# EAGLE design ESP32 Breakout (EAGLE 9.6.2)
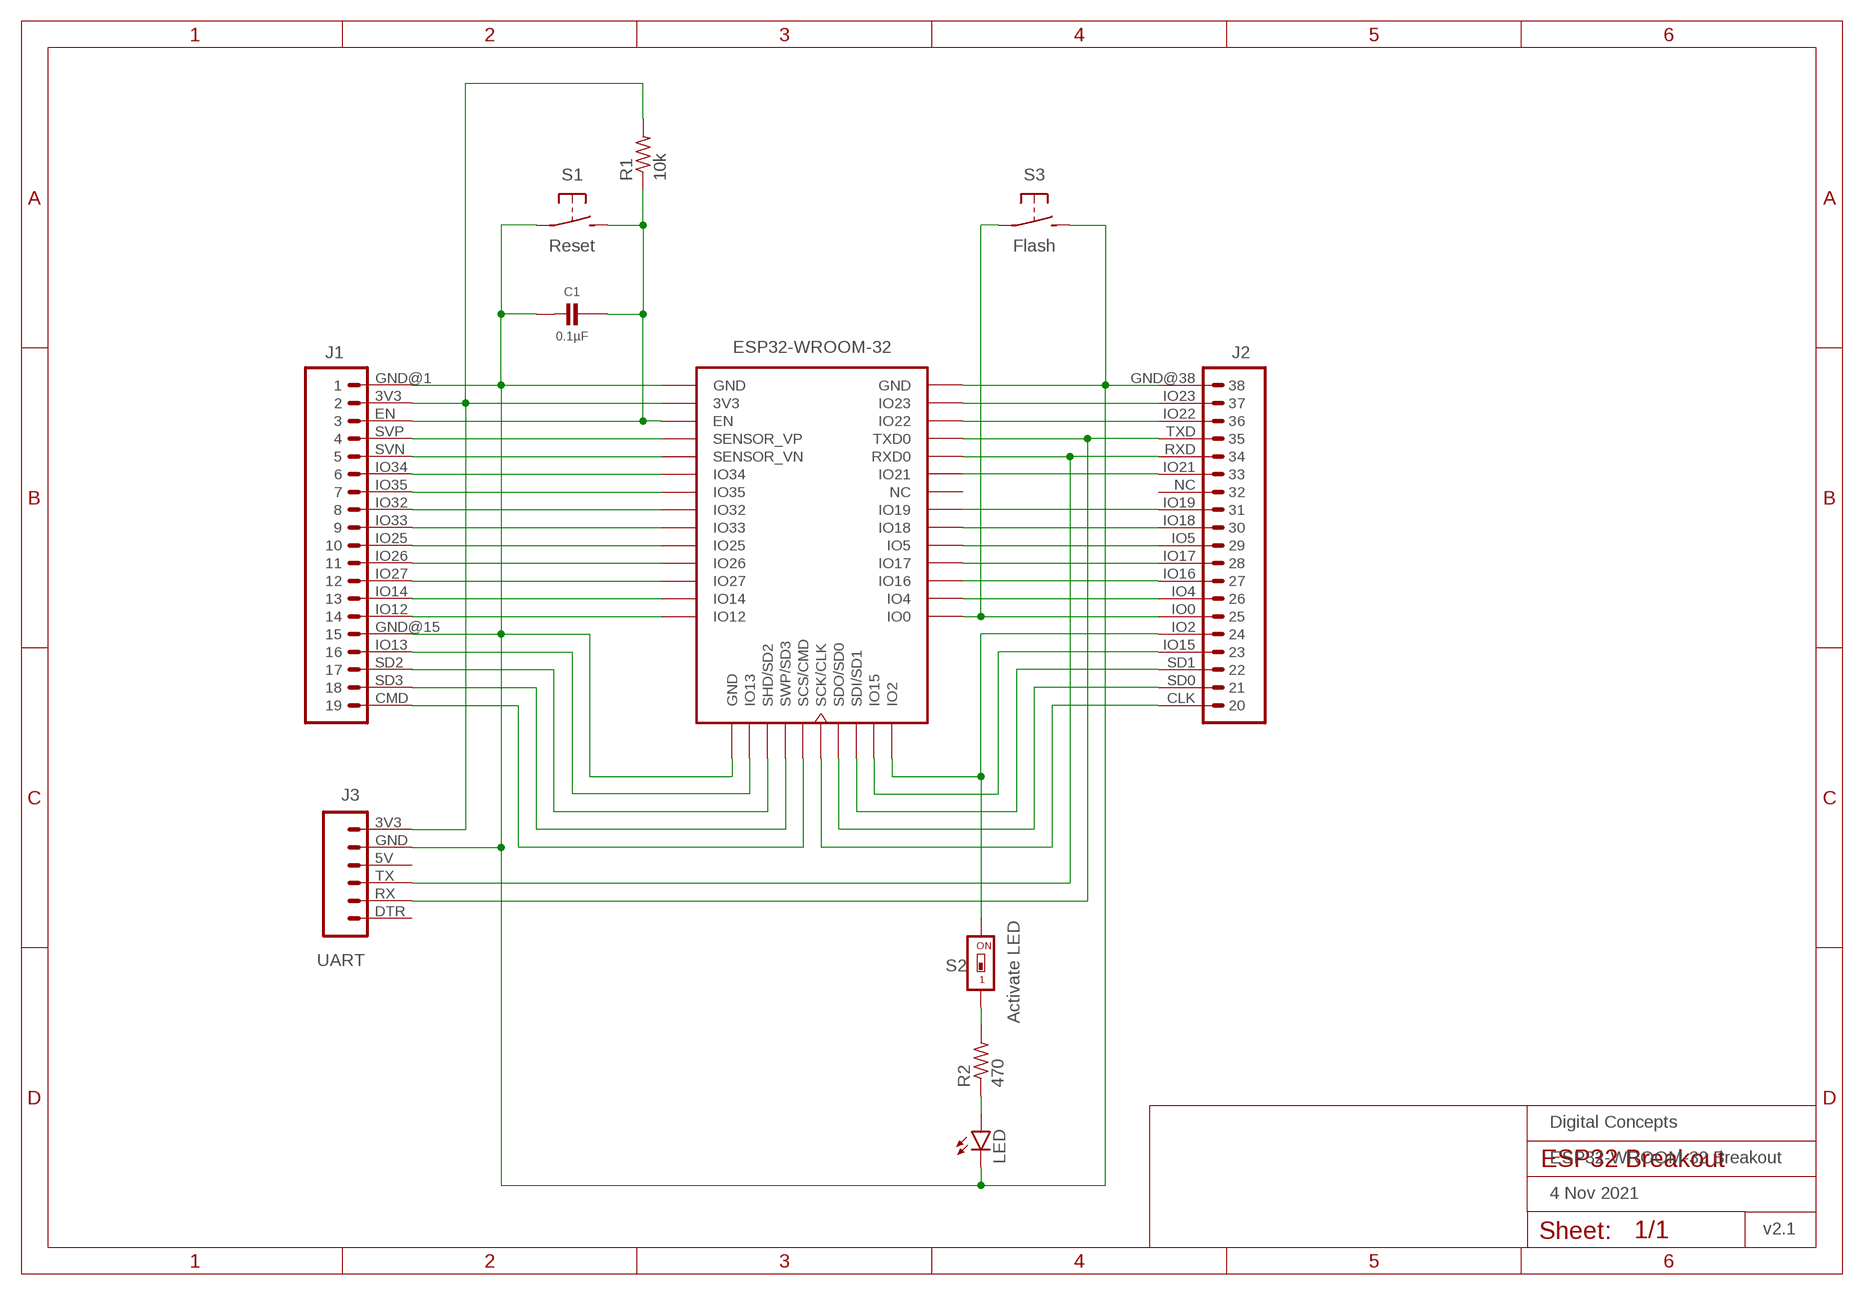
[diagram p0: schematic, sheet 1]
FRAME1 (A4L-LOC): DATE: 4 Nov 2021; OWNER: Digital Concepts; TITLE: ESP32-WROOM-32 Breakout; VERSION: v2.1

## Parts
C1  0.1µF  CAPACITOR-0805  [C0805]
J1  HEADER-1X19-ESP32-L  [CONN_19-ESP32-L]
J2  HEADER-1X19-ESP32-R  [CONN_19-ESP32-R]
J3  UART  HEADER-1X6-UART  [CONN_06-UART]
LED  LEDCHIP-LED0805  [CHIP-LED0805]
R1  10k  RESISTOR-VIA-2  [R0805-VIA-2]
R2  470  RESISTORR0805  [R0805]
S1  Reset  SWITCH-MOMENTARY-2-PIN  [SWITCH-2-PAD]
S2  Activate LED  SWITCH-DIP-SWS001  [SMD-001]
S3  Flash  SWITCH-MOMENTARY-2-PIN  [SWITCH-2-PAD]
U1  ESP32-WROOM-32  ESP32-WROOM-32-CHIP  [ESP32-WROOM-32]

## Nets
GND: C1.2 J1.GND@1 J1.GND@15 J2.GND@38 J3.GND LED.C S1.P$1(P) S3.P$2(S) U1.GND@1(GND) U1.GND@15(GND) U1.GND@38(GND) U1.TP(GND) U1.TP@P1(GND) U1.TP@P2(GND) U1.TP@P3(GND) U1.TP@P4(GND) U1.TP@P5(GND) U1.TP@P6(GND) U1.TP@P7(GND) U1.TP@P8(GND) U1.TP@P9(GND) U1.TP@V1(GND) U1.TP@V2(GND) U1.TP@V3(GND) U1.TP@V4(GND) U1.TP@V5(GND) U1.TP@V6(GND) U1.TP@V7(GND) U1.TP@V8(GND) U1.TP@V9(GND) U1.TP@V10(GND) U1.TP@V11(GND) U1.TP@V12(GND) U1.TP@VP5(GND)
N$1: R2.2 S2.1
N$2: J1.SVP U1.SENSOR_VP
N$3: C1.1 J1.EN R1.1 S1.P$2(S) U1.EN
N$4: J1.IO32 U1.IO32
N$5: J1.SVN U1.SENSOR_VN
N$6: J1.IO34 U1.IO34
N$7: J1.IO35 U1.IO35
N$8: LED.A R2.1
N$13: J2.IO19 U1.IO19
N$14: J2.IO17 U1.IO17
N$15: J1.CMD U1.CMD(SCS/CMD)
N$16: J2.IO18 U1.IO18
N$17: J2.IO22 U1.IO22
N$18: J2.IO15 U1.IO15
N$19: J2.CLK U1.CLK(SCK/CLK)
N$20: J2.SD0 U1.SD0(SDO/SD0)
N$21: J2.SD1 U1.SD1(SDI/SD1)
N$22: J2.IO23 U1.IO23
N$23: J2.IO2 S2.2 U1.IO2
N$24: J2.IO0 S3.P$1(P) U1.IO0
N$25: J2.IO4 U1.IO4
N$26: J2.IO16 U1.IO16
N$28: J2.IO5 U1.IO5
N$31: J2.RXD J3.TX U1.RXD0
N$32: J2.TXD J3.RX U1.TXD0
N$35: J2.IO21 U1.IO21
N$36: J1.IO33 U1.IO33
N$38: J1.IO25 U1.IO25
N$39: J1.IO26 U1.IO26
N$40: J1.IO27 U1.IO27
N$41: J1.IO14 U1.IO14
N$42: J1.IO12 U1.IO12
N$43: J1.SD2 U1.SD2(SHD/SD2)
N$45: J1.IO13 U1.IO13
N$46: J1.SD3 U1.SD3(SWP/SD3)
VCC: J1.3V3 J3.3V3 R1.2 R1.2@VIA U1.3V3
Unconnected: J2.NC J3.5V J3.DTR U1.NC

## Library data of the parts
C1 = digitalconcepts:CAPACITOR-0805: 0805 Capacitor
J1 = digitalconcepts:HEADER-1X19-ESP32-L: ESP32 Left 19-Pin Header
J2 = digitalconcepts:HEADER-1X19-ESP32-R: ESP32 Right 19-Pin Header
J3 = digitalconcepts:HEADER-1X6-UART: Single Row 6-Pin UART Header
LED = digitalconcepts:LED: LED
R1 = digitalconcepts:RESISTOR-VIA-2: Resistor with via on Pad 2
R2 = digitalconcepts:RESISTOR: Resistor; SPICEPREFIX: R
S1 S3 = digitalconcepts:SWITCH-MOMENTARY-2-PIN: 2 Pin Momentary Switch
S2 = digitalconcepts:SWITCH-DIP-SWS001: SMD Dip Switch 1 pol.
U1 = digitalconcepts:ESP32-WROOM-32-CHIP: ESP32-WROOM-32 Chip

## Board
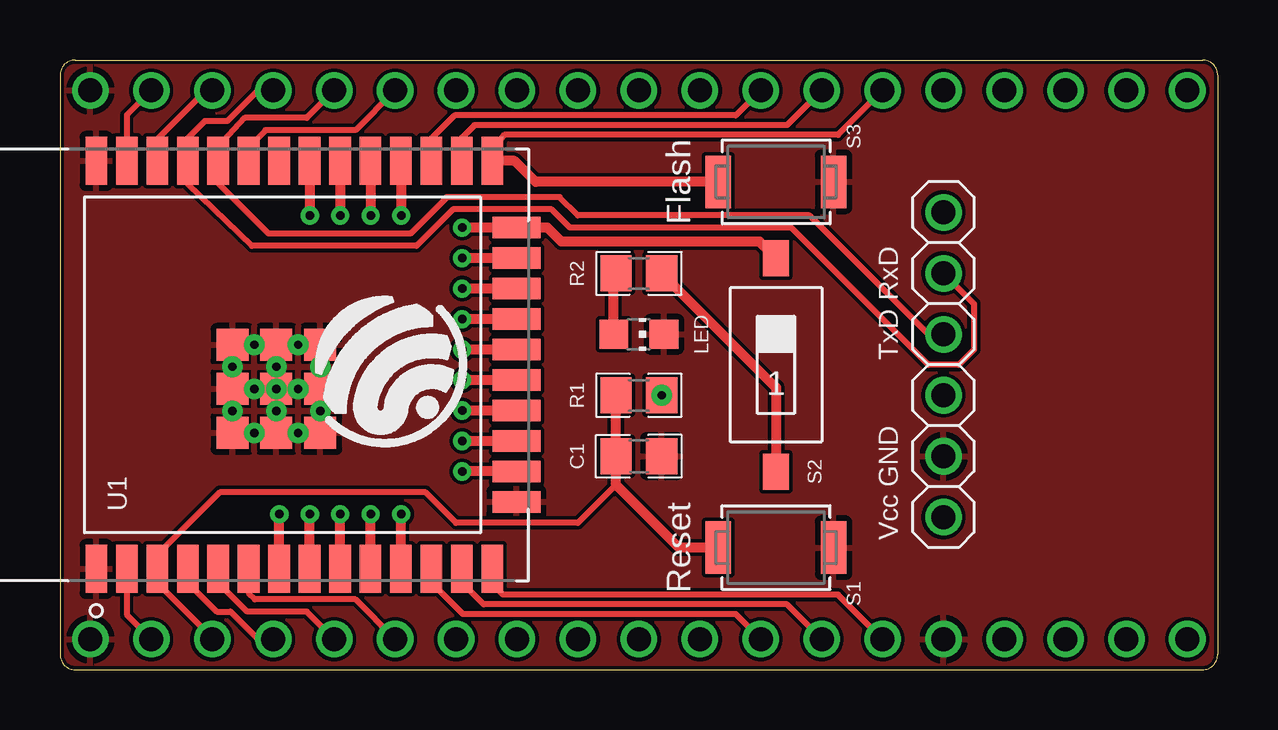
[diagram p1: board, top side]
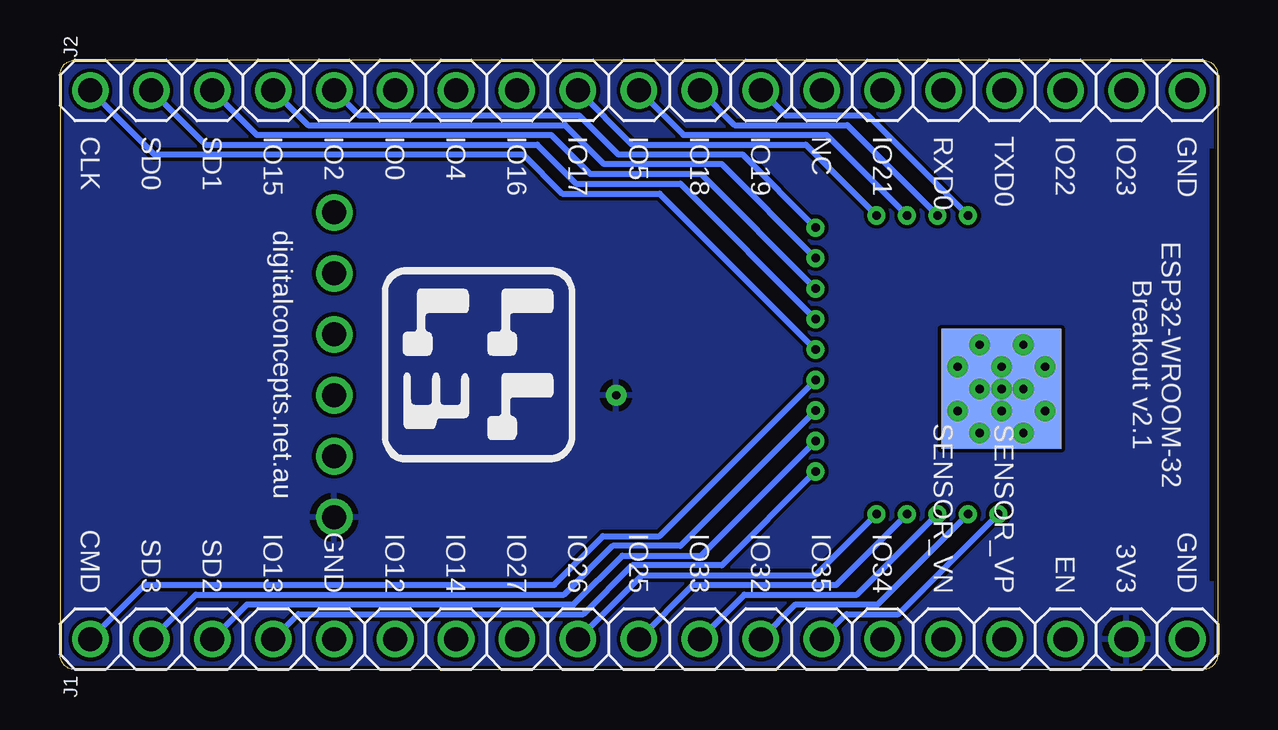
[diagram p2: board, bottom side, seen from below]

Size 48.26 x 25.4 mm. Coordinates in mm from the lower left corner, seen from the top.
Outline: 0,24.77 0,0.64 arc90 0.64,0 47.62,0 arc90 48.26,0.64 48.26,24.77 arc90 47.62,25.4 0.64,25.4 arc90 0,24.77
Copper layers (1*16): Top 0.035mm / dielectric 1.5mm / Bottom 0.035mm
Design rules "default *": minimum track width 6mil, minimum drill 0.35mm, track to track 6mil, track to pad 6mil, pad to pad 6mil, via to via 6mil, smd to smd 6mil, copper to edge 6mil, drill to drill 6mil, minimum pad ring 10mil, minimum via ring 8mil, stop-mask expansion 4mil, vias tented up to drill 0mil, thermal gap 10mil

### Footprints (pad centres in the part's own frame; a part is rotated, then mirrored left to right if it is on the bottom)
C0805 = smd 1.3 x 1.5: 1 -0.95,0; 2 0.95,0
CONN_19-ESP32-L = drill 1 pad 1.524: 3V3 43.18,0; CMD 0,0; EN 40.64,0; GND@1 45.72,0; GND@15 10.16,0; IO12 12.7,0; IO13 7.62,0; IO14 15.24,0; IO25 22.86,0; IO26 20.32,0; IO27 17.78,0; IO32 27.94,0; IO33 25.4,0; IO34 33.02,0; IO35 30.48,0; SD2 5.08,0; SD3 2.54,0; SVN 35.56,0; SVP 38.1,0
CONN_19-ESP32-R = drill 1 pad 1.524: CLK 0,0; GND@38 45.72,0; IO0 12.7,0; IO2 10.16,0; IO4 15.24,0; IO5 22.86,0; IO15 7.62,0; IO16 17.78,0; IO17 20.32,0; IO18 25.4,0; IO19 27.94,0; IO21 33.02,0; IO22 40.64,0; IO23 43.18,0; NC 30.48,0; RXD 35.56,0; SD0 2.54,0; SD1 5.08,0; TXD 38.1,0
CONN_06-UART = drill 1 pad 1.524: 3V3 12.7,0; 5V 7.62,0; DTR 0,0; GND 10.16,0; RX 2.54,0; TX 5.08,0
CHIP-LED0805 = smd 1.2 x 1.2: A 0,-1.05; C 0,1.05
R0805-VIA-2 = smd 1.3 x 1.5: 1 -0.95,0; 2 0.95,0 | drill 0.35 pad 0.61: 2@VIA 0.95,0
R0805 = smd 1.3 x 1.5: 1 -0.95,0; 2 0.95,0
SWITCH-2-PAD = smd 1.067 x 2.184: P$1 -2.4,0; P$2 2.4,0
SMD-001 = smd 1.1 x 1.5: 1 0,-4.45; 2 0,4.45
ESP32-WROOM-32 = smd 2 x 0.9: 3V3 -8.5,6.74; EN -8.5,5.47; GND@1 -8.5,8.01; GND@38 8.5,8.01; IO0 8.5,-8.5; IO4 8.5,-7.23; IO5 8.5,-3.42; IO12 -8.5,-8.5; IO14 -8.5,-7.23; IO16 8.5,-5.96; IO17 8.5,-4.69; IO18 8.5,-2.15; IO19 8.5,-0.88; IO21 8.5,1.66; IO22 8.5,5.47; IO23 8.5,6.74; IO25 -8.5,-3.42; IO26 -8.5,-4.69; IO27 -8.5,-5.96; IO32 -8.5,-0.88; IO33 -8.5,-2.15; IO34 -8.5,1.66; IO35 -8.5,0.39; NC 8.5,0.39; RXD0 8.5,2.93; SENSOR_VN -8.5,2.93; SENSOR_VP -8.5,4.2; TXD0 8.5,4.2 | smd 0.9 x 2: CLK 0.635,-9.5; CMD -0.635,-9.5; GND@15 -5.715,-9.5; IO2 5.715,-9.5; IO13 -4.445,-9.5; IO15 4.445,-9.5; SD0 1.905,-9.5; SD1 3.175,-9.5; SD2 -3.175,-9.5; SD3 -1.905,-9.5 | smd 5 x 5 bottom: TP -1,0.51 | smd 1.33 x 1.33: TP@P1 -2.835,2.335; TP@P2 -1,2.335; TP@P3 0.835,2.335; TP@P4 -2.835,0.51; TP@P5 -1,0.51; TP@P6 0.835,0.51; TP@P7 -2.835,-1.325; TP@P8 -1,-1.325; TP@P9 0.835,-1.325 | drill 0.35 pad 0.406: TP@V1 -1.917,2.335; TP@V2 -0.083,2.335; TP@V3 -2.835,1.423; TP@V4 -1,1.423; TP@V5 0.835,1.423; TP@V6 -1.917,0.51; TP@V7 -0.083,0.51; TP@V8 -2.835,-0.403; TP@V9 -1,-0.403; TP@V10 0.835,-0.403; TP@V11 -1.917,-1.325; TP@V12 -0.083,-1.325; TP@VP5 -1,0.51

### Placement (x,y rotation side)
C1  24.13,8.89 0 top
J1  46.99,1.27 0 bottom
J2  46.99,24.13 0 bottom
J3  36.83,19.05 270 top
LED  24.13,13.97 270 top
R1  24.13,11.43 0 top
R2  24.13,16.51 0 top
S1  29.85,5.08 180 top
S2  29.85,12.7 0 top
S3  29.85,20.32 0 top
U1  9.53,12.7 90 top

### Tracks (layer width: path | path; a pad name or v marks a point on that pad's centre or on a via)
GND
  pour Top (rank 3): -1.27,26.67 49.53,26.67 49.53,-1.4 -1.27,-1.4
N$1
  Top 0.406: R2.2 29.85,11.75 S2.1
N$2
  Top 0.254: U1.SENSOR_VP 5.32,3.62 6.54,2.41 7.11,2.41 8.25,1.27 J1.SVP
N$3
  Top 0.254: J1.EN 6.35,1.33 4.05,3.62 U1.EN 4.05,4.78 6.66,7.38 15.24,7.38 16.51,6.11 21.59,6.11 23.18,7.7
  Top 0.406: R1.1 C1.1 23.18,7.7 25.8,5.08 S1.P$2
N$4  (via drill 0.35)
  Top 0.406: U1.IO32 10.41,6.47 v10.41,6.48
  Bottom 0.254: v10.41,6.48 14.17,2.72 17.6,2.72 J1.IO32
N$5
  Top 0.254: U1.SENSOR_VN 6.6,3.62 7.81,2.41 10.29,2.41 J1.SVN
N$6
  Top 0.254: U1.IO34 7.87,3.18 8.13,2.92 12.32,2.92 J1.IO34
N$7  (via drill 0.35)
  Top 0.406: U1.IO35 9.14,6.47 v9.14,6.48
  Bottom 0.254: v9.14,6.48 13.31,2.31 15.47,2.31 J1.IO35
N$8
  Top 0.406: LED.A 23.08,16.41 R2.1
N$13  (via drill 0.35)
  Top 0.406: U1.IO19 v10.41,18.92
  Bottom 0.254: v10.41,18.92 14.58,23.09 18.01,23.09 J2.IO19
N$14  (via drill 0.35)
  Top 0.406: U1.IO17 14.21,18.93 v14.22,18.92
  Bottom 0.254: v14.22,18.92 17.17,21.87 24.41,21.87 J2.IO17
N$15  (via drill 0.35)
  Top 0.406: U1.CMD v16.76,12.07
  Bottom 0.254: J1.CMD 44.73,3.53 27.66,3.53 25.63,5.56 23.27,5.56 v16.76,12.07
N$16  (via drill 0.35)
  Top 0.406: U1.IO18 11.68,18.93 v11.68,18.92
  Bottom 0.254: v11.68,18.92 15.44,22.68 20.14,22.68 J2.IO18
N$17
  Top 0.254: U1.IO22 4.05,22.09 6.1,24.13 J2.IO22
N$18  (via drill 0.35)
  Top 0.406: U1.IO15 v16.76,17.14
  Bottom 0.254: v16.76,17.14 20.68,21.06 25.58,21.06 27.2,22.68 37.92,22.68 J2.IO15
N$19  (via drill 0.35)
  Top 0.406: U1.CLK v16.76,13.34
  Bottom 0.254: v16.76,13.34 23.27,19.84 27.33,19.84 28.96,21.46 44.32,21.46 J2.CLK
N$20  (via drill 0.35)
  Top 0.406: U1.SD0 v16.76,14.61
  Bottom 0.254: v16.76,14.61 22.4,20.24 26.75,20.24 28.37,21.87 42.19,21.87 J2.SD0
N$21  (via drill 0.35)
  Top 0.406: U1.SD1 v16.76,15.88
  Bottom 0.254: v16.76,15.88 21.54,20.65 26.16,20.65 27.79,22.28 40.06,22.28 J2.SD1
N$22
  Top 0.254: J2.IO23 2.79,23.11 U1.IO23
N$23  (via drill 0.35)
  Top 0.406: v16.76,18.41 U1.IO2 20.32,18.41 20.9,17.83 29.16,17.83 S2.2
  Bottom 0.254: v16.76,18.41 19.81,21.46 24.99,21.46 26.62,23.09 35.79,23.09 J2.IO2
N$24
  Top 0.254: U1.IO0 18.03,21.64 18.51,22.28 32.44,22.28 J2.IO0
  Top 0.406: S3.P$1 19.82,20.32 18.95,21.2 U1.IO0
N$25
  Top 0.254: U1.IO4 16.75,22.17 17.27,22.68 30.3,22.68 J2.IO4
N$26
  Top 0.254: U1.IO16 15.48,22.13 16.44,23.09 28.17,23.09 J2.IO16
N$28  (via drill 0.35)
  Top 0.406: U1.IO5 v12.95,18.92
  Bottom 0.254: v12.95,18.92 16.31,22.28 22.28,22.28 J2.IO5
N$31
  Top 0.254: J2.RXD 10.29,22.99 7.71,22.99 6.6,21.78 U1.RXD0 6.6,20.25 8.69,18.16 14.61,18.16 16.13,19.68 20.83,19.68 21.59,18.92 31.24,18.92 36.2,13.97 J3.TX
N$32
  Top 0.254: J2.TXD 8.25,24.13 6.98,22.85 6.04,22.85 5.32,22.14 U1.TXD0 5.32,20.24 8.01,17.65 14.86,17.65 16.38,19.18 20.5,19.18 21.26,18.41 30.48,18.41 36.2,12.7 37.47,12.7 38.1,13.34 38.1,15.24 J3.RX
N$35
  Top 0.254: U1.IO21 7.87,21.78 8.57,22.48 12.32,22.48 J2.IO21
N$36  (via drill 0.35)
  Top 0.406: U1.IO33 11.68,6.47 v11.68,6.48
  Bottom 0.254: v11.68,6.48 15.04,3.12 19.74,3.12 J1.IO33
N$38  (via drill 0.35)
  Top 0.406: U1.IO25 12.95,6.47 v12.95,6.48
  Bottom 0.254: v12.95,6.48 15.9,3.53 21.87,3.53 J1.IO25
N$39  (via drill 0.35)
  Top 0.406: U1.IO26 14.21,6.47 v14.22,6.48
  Bottom 0.254: v14.22,6.48 16.76,3.94 24,3.94 J1.IO26
N$40
  Top 0.254: U1.IO27 15.48,3.62 16.8,2.31 28.17,2.31 J1.IO27
N$41
  Top 0.254: U1.IO14 16.75,3.62 17.66,2.72 30.3,2.72 J1.IO14
N$42
  Top 0.254: U1.IO12 18.03,3.57 18.47,3.12 32.44,3.12 J1.IO12
N$43  (via drill 0.35)
  Top 0.406: U1.SD2 v16.76,9.53
  Bottom 0.254: v16.76,9.53 21.54,4.75 24.82,4.75 26.85,2.72 40.46,2.72 J1.SD2
N$45  (via drill 0.35)
  Top 0.406: U1.IO13 v16.76,8.25
  Bottom 0.254: v16.76,8.25 20.68,4.34 24.41,4.34 26.44,2.31 38.33,2.31 J1.IO13
N$46  (via drill 0.35)
  Top 0.406: U1.SD3 v16.76,10.8
  Bottom 0.254: v16.76,10.8 22.4,5.16 25.22,5.16 27.25,3.12 42.6,3.12 J1.SD3
VCC
  Top 0.254: U1.3V3 2.79,2.29 J1.3V3
  pour Bottom (rank 3): -0.63,26.04 48.89,26.04 48.89,-0.63 -0.63,-0.63

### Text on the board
tPlace: RxD | TxD | GND | Vcc
bPlace: GND | IO23 | IO22 | TXD0 | RXD0 | IO21 | NC | IO19 | IO18 | IO5 | IO17 | IO16 | IO4 | IO0 | IO2 | IO15 | SD1 | SD0 | CLK | ESP32-WROOM-32 / Breakout v2.1 | digitalconcepts.net.au | GND | 3V3 | EN | SENSOR_VP | SENSOR_VN | IO34 | IO35 | IO32 | IO33 | IO25 | IO26 | IO27 | IO14 | IO12 | GND | IO13 | SD2 | SD3 | CMD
